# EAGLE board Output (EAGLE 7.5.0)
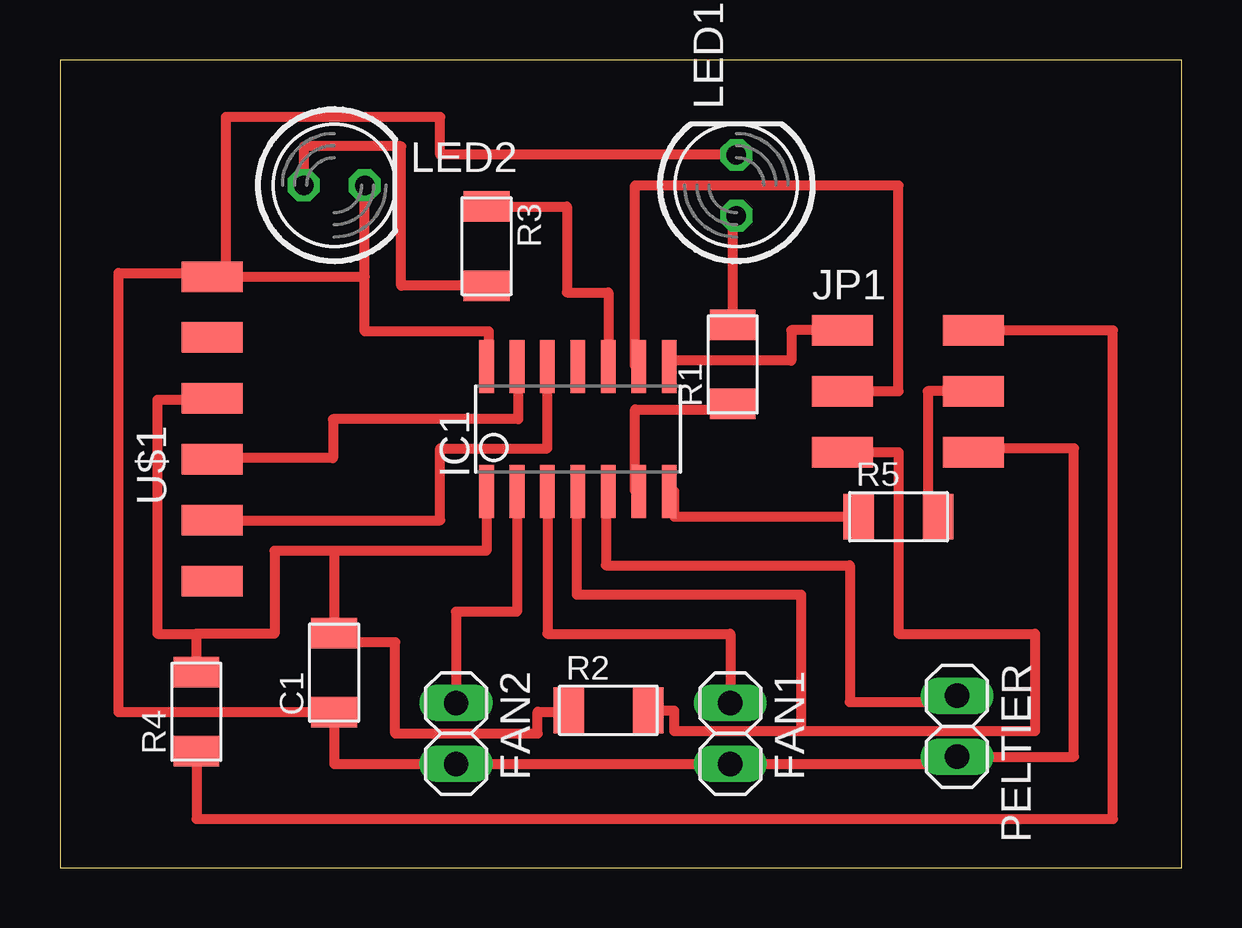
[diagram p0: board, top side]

Size 46.76 x 33.67 mm. Coordinates in mm from the lower left corner, seen from the top.
Outline: 0,0 46.76,0 46.76,33.67 0,33.67 0,0
Copper layers (1*16): Top 0.035mm / dielectric 1.5mm / Bottom 0.035mm
Design rules "default *": minimum track width 16mil, minimum drill 24mil, track to track 16mil, track to pad 16mil, pad to pad 16mil, via to via 16mil, smd to smd 16mil, copper to edge 40mil, drill to drill 8mil, minimum pad ring 10mil, minimum via ring 8mil, stop-mask expansion 4mil, vias tented up to drill 0mil, thermal gap 10mil

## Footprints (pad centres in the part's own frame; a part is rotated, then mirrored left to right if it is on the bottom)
C1206FAB = smd 1.27 x 1.905: 1 -1.651,0; 2 1.651,0
1X02 = drill 1.016 long: 1 -1.27,0; 2 1.27,0
SOIC14 = smd 0.61 x 2.21: 1 -3.81,-2.603; 2 -2.54,-2.603; 3 -1.27,-2.603; 4 0,-2.603; 5 1.27,-2.603; 6 2.54,-2.603; 7 3.81,-2.603; 8 3.81,2.603; 9 2.54,2.603; 10 1.27,2.603; 11 0,2.603; 12 -1.27,2.603; 13 -2.54,2.603; 14 -3.81,2.603
2X03SMD = smd 2.54 x 1.27: 1 -2.54,2.54; 2 2.92,2.54; 3 -2.54,0; 4 2.92,0; 5 -2.54,-2.54; 6 2.92,-2.54
LED5MM = drill 0.813 octagon: A -1.27,0; K 1.27,0
R1206FAB = smd 1.27 x 1.905: 1 -1.651,0; 2 1.651,0
1X06SMD = smd 2.54 x 1.27: 1 0,6.35; 2 0,3.81; 3 0,1.27; 4 0,-1.27; 5 0,-3.81; 6 0,-6.35

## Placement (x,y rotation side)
C1  1uF  [C1206FAB]  11.43,8.13 90 top
FAN1  [1X02]  27.94,5.59 270 top
FAN2  [1X02]  16.51,5.59 270 top
IC1  ATTINY44-SSU  [SOIC14]  21.59,18.29 0 top
JP1  [2X03SMD]  35.15,19.86 0 top
LED1  [LED5MM]  28.19,28.45 90 top
LED2  [LED5MM]  11.43,28.45 0 top
PELTIER  [1X02]  37.39,5.89 270 top
R1  290  [R1206FAB]  28.04,20.98 90 top
R2  10k  [R1206FAB]  22.86,6.55 0 top
R3  290  [R1206FAB]  17.78,25.91 270 top
R4  0  [R1206FAB]  5.69,6.5 90 top
R5  0  [R1206FAB]  34.95,14.63 0 top
U$1  FTDI-SMD-HEADER  [1X06SMD]  6.35,18.29 0 top

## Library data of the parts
C1 IC1 JP1 R1-R5 U$1 = fab
FAN1 FAN2 PELTIER = pinhead
LED1 LED2 = led

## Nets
N$1: C1.1 FAN1.2 FAN2.2 IC1.14 JP1.6 LED1.K LED2.K PELTIER.2 U$1.1
N$2: C1.2 IC1.1 R2.1 R4.2 U$1.3
N$3: IC1.6 R1.1
N$4: LED1.A R1.2
N$5: LED2.A R3.2
N$6: FAN1.1 IC1.3
N$7: IC1.8 JP1.1
N$8: IC1.10 R3.1
N$9: IC1.7 R5.1
N$10: IC1.13 U$1.4
N$11: IC1.12 U$1.5
N$12: IC1.9 JP1.3
N$13: IC1.4 JP1.5 R2.2
N$14: IC1.5 PELTIER.1
N$15: FAN2.1 IC1.2
N$16: JP1.2 R4.1
N$17: JP1.4 R5.2

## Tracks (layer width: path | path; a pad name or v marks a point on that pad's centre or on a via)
N$1
  Top 0.406: IC1.14 17.88,20.89 17.88,22.35 12.7,22.35 12.7,24.64 | 12.7,24.64 LED2.K | U$1.1 6.91,24.64 | 6.91,24.64 7.32,24.64 | 7.32,24.64 12.7,24.64 | LED1.K 15.85,29.72 15.85,31.29 6.91,31.29 6.91,24.64 | 7.32,24.64 7.32,24.79 2.44,24.79 2.44,6.48 C1.1 11.43,4.32 FAN2.2 FAN1.2 37.39,4.32 PELTIER.2 42.27,4.62 42.27,17.48 38.07,17.48 JP1.6
N$2
  Top 0.406: IC1.1 17.78,13.21 11.43,13.21 | 11.43,13.21 C1.2 11.43,9.4 13.97,9.4 13.97,5.59 19.91,5.59 19.91,6.5 21.21,6.5 R2.1 | 11.43,13.21 8.94,13.21 8.94,9.75 5.69,9.75 | U$1.3 6.35,19.51 4.06,19.51 4.06,9.75 5.69,9.75 | R4.2 5.69,9.75
N$3
  Top 0.406: IC1.6 23.98,15.68 23.98,19.1 28.04,19.1 R1.1
N$4
  Top 0.406: LED1.A 28.04,27.18 R1.2
N$5
  Top 0.406: R3.2 14.22,24.26 14.22,30.07 10.16,30.07 LED2.A
N$6
  Top 0.406: IC1.3 20.32,9.75 27.94,9.75 FAN1.1
N$7
  Top 0.406: JP1.1 30.48,22.4 30.48,21.13 25.4,21.13 IC1.8
N$8
  Top 0.406: R3.1 21.13,27.56 21.13,23.98 22.86,23.98 IC1.10
N$9
  Top 0.406: IC1.7 25.6,15.68 25.6,14.63 R5.1
N$10
  Top 0.406: IC1.13 19.1,20.89 19.1,18.69 11.38,18.69 11.38,17.07 6.35,17.07 U$1.4
N$11
  Top 0.406: U$1.5 15.85,14.48 15.85,17.48 20.32,17.48 IC1.12
N$12
  Top 0.406: IC1.9 23.98,20.89 23.98,28.45 34.95,28.45 34.95,19.86 JP1.3
N$13
  Top 0.406: 30.89,5.69 40.64,5.69 40.64,9.75 34.95,9.75 34.95,17.32 JP1.5 | 30.89,5.69 25.6,5.69 25.6,6.55 R2.2 | IC1.4 21.54,15.68 21.54,11.38 30.89,11.38 30.89,5.69
N$14
  Top 0.406: IC1.5 22.76,15.68 22.76,12.6 32.92,12.6 32.92,6.91 37.39,6.91 PELTIER.1
N$15
  Top 0.406: IC1.2 19.05,10.67 16.51,10.67 FAN2.1
N$16
  Top 0.406: R4.1 5.69,2.03 43.89,2.03 43.89,22.4 JP1.2
N$17
  Top 0.406: JP1.4 36.17,19.86 36.17,14.63 R5.2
